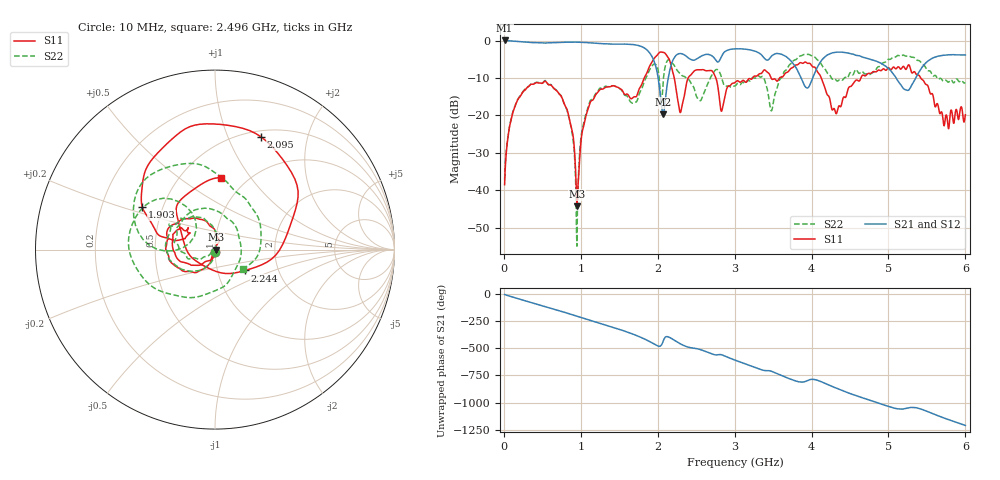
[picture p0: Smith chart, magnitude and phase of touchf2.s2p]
!  15/09/2025  16:04:16
! Ref Plane: 0.000 mm
# MHZ S MA R  50
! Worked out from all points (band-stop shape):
!   1001 points, 10 MHz to 6 GHz, reference 50 ohm
!   highest |S21| = 0.02 dB at 10 MHz (marker M1); lowest = -19.7 dB at 2.071 GHz (marker M2)
!   |S21| within 3 dB of the highest: start of sweep to 1.883 GHz; 2.873 GHz to 3.284 GHz (411.9 MHz wide, 13.4 % of centre)
!   lowest |S11| = -44.3 dB at 950.4 MHz (marker M3), VSWR 1.01, Z = 50.6 + j0.0472 ohm
!   |S11| at or under -10 dB: start of sweep to 1.825 GHz; 4.126 GHz to 4.642 GHz (515.4 MHz wide, 11.8 % of centre); 5.419 GHz to end of sweep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
!   |S22| runs from -54.9 to -3.7 dB; largest |S21 - S12| = 0.012
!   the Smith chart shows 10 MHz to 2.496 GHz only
!   S11 on the Smith chart (normalised r, x): 10 MHz: 1.00, -0.02; 1.903 GHz: 0.38, +0.23; 2.095 GHz: 0.57, +1.33; 2.244 GHz: 1.36, -0.33; 2.496 GHz: 0.76, +0.73
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10  0.01192 -81.4  1.002 -2.2  0.9954 -2.1  0.01391 -82.9
165.74  0.1499 -126.9  0.9761 -36.6  0.9709 -36.8  0.1515 -129.1
543.11  0.2852 154.8  0.9253 -114.7  0.9205 -114.8  0.2911 151.7
830.63  0.1118 91.3  0.9509 -175.6  0.947 -175.7  0.1082 90.5
950.43  0.00611 4.4  0.9512 157.8  0.9466 157.7  0.0018 -159.7
1010.33  0.05309 -112.0  0.947 144.5  0.9418 144.4  0.05747 -140.4
1585.37  0.1904 141.6  0.8951 16.1  0.892 16.1  0.184 65.9
1902.84  0.4707 149.6  0.6664 -79.2  0.6636 -79.4  0.4215 -154.8
2010.66  0.6725 108.6  0.2923 -119.8  0.2911 -119.9  0.373 130.9
2070.56  0.6948 80.5  0.1039 -75.2  0.1035 -75.1  0.2771 -178.3
2094.52  0.6785 67.7  0.1438 -39.2  0.1436 -39.1  0.4361 167.6
2244.27  0.2049 -34.5  0.6419 -77.5  0.6385 -77.7  0.4128 86.8
2495.85  0.4031 85.2  0.5592 -140.8  0.5566 -140.9  0.1908 -34.2
3005  0.275 -18.6  0.7744 111.6  0.7703 111.3  0.2476 55.2
3310.49  0.3536 -105.3  0.6866 32.4  0.6848 32.2  0.3379 -27.2
3687.86  0.3779 158.9  0.5897 -53.4  0.5879 -53.6  0.429 -120.2
4005.33  0.4553 30.4  0.2998 -65.8  0.2999 -66.1  0.6267 127.1
4436.61  0.1735 75.9  0.692 -179.9  0.6889 180.0  0.3224 85.5
5005.66  0.431 -165.3  0.4155 42.1  0.414 42.0  0.561 38.3
5245.26  0.4473 70.7  0.2158 26.8  0.215 26.7  0.6236 -11.5
5586.69  0.1688 -100.6  0.5911 -26.1  0.5877 -25.9  0.336 -70.3
6000  0.102 7.3  0.6409 -132.1  0.6374 -132.0  0.2741 -100.5
